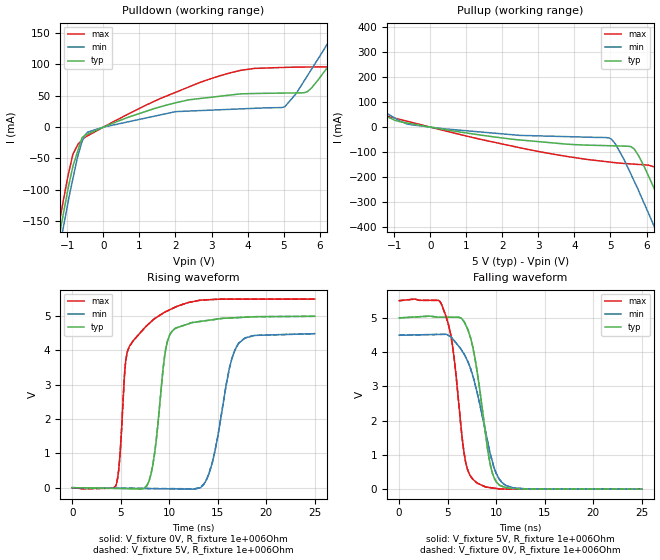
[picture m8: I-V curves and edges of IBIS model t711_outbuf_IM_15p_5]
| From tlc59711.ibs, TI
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|   t711_outbuf 5V Model with
|   1M ohm and 15 pf load during VT transient
[Model] t711_outbuf_IM_15p_5
Model_type   Output
Polarity   Non-Inverting
Vmeas = 2.5
Vref = 2.5
Cref = 15pF
Rref = 50
|   typ   min   max
|   (nom PVT)   (Fast PVT)   (slow PVT)
|   ON state : BUFFER OUTPUT TURNED HIGH
C_comp   1.98646E-12   1.61466E-12   2.27029E-12
|   OFF state: BUFFER OUTPUT TURNED LOW
|C_comp   1.92343E-12   1.92343E-12   1.92343E-12
| Where   nom PVT is  Nominal Process, 5V, 90C
|   Fast PVT is Strong Process, 4.5V, -40C
|   Slow PVT is Weak Process, 5.5V, 150C
|   C_comp - from L-C Tank method, L = 1nH, peak frequency
| variable   typ   min   max
[Voltage Range]   5   4.5   5.5
|Operating Temperature Range
|   25   85   -40
|Junction Temperature Range
[Temperature Range]   90   150   -40
[Pullup Reference]   5   4.5   5.5
[Pulldown Reference]   0   0   0
[Power Clamp Reference]   5   4.5   5.5
[GND Clamp Reference]   0   0   0
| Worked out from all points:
|   slope of the pulldown table from 0 to 0.75 V, typ, clamps not added: 44.2 ohm
|   slope of the pullup table from 0 to 0.75 V, typ, clamps not added: 42.1 ohm
|   falling waveform, V_fixture 5V, R_fixture 1e+006Ohm: 20-80 % time 1.52ns typ, 2.26ns min, 1.29ns max; typ from 5 V to 0.001 V
|   rising waveform, V_fixture 0V, R_fixture 1e+006Ohm: 20-80 % time 1.13ns typ, 1.72ns min, 1.69ns max; typ from 0.001 V to 5 V
|   rising waveform, V_fixture 5V, R_fixture 1e+006Ohm: 20-80 % time 1.13ns typ, 1.73ns min, 1.69ns max; typ from 0.001 V to 5 V
|   falling waveform, V_fixture 0V, R_fixture 1e+006Ohm: 20-80 % time 1.52ns typ, 2.26ns min, 1.29ns max; typ from 5 V to 0.001 V
[Pulldown]
|   Voltage   I(typ)   I(min)   I(max)
-5V       -1.595A    -1.55A     -1.658A
-1.243V   -178.9mA   -200.3mA   -159.4mA
-1.11V    -138mA     -159.3mA   -116.4mA
-840.5mV  -61.25mA   -80.66mA   -42.53mA
-598.2mV  -17.61mA   -23.71mA   -21.08mA
-419.1mV  -10.56mA   -7.658mA   -13.18mA
2.678V    45.63mA    26.39mA    71.32mA
5.023V    54.34mA    32.3mA     95.27mA
5.663V    56.68mA    82.24mA    95.89mA
6.506V    119.4mA    161mA      104mA
7.553V    207mA      262.9mA    172mA
9.985V    423.5mA    510mA      347.6mA
[Pullup]
|   Voltage   I(typ)   I(min)   I(max)
-5V       352.5mA    416.3mA    271.4mA
-2.121V   116.7mA    142.1mA    82.16mA
-663.7mV  17.22mA    13.61mA    24.41mA
2.374V    -49.89mA   -31.61mA   -79mA
4.987V    -74.39mA   -44.7mA    -139.8mA
5.137V    -74.98mA   -67.29mA   -142.3mA
5.663V    -88.31mA   -217.5mA   -148.1mA
6.226V    -250mA     -402.2mA   -159.9mA
6.358V    -295.2mA   -447.7mA   -174.7mA
6.712V    -419.1mA   -571.8mA   -288.4mA
7.056V    -542.9mA   -693.1mA   -417.9mA
9.985V    -1.675A    -1.779A    -1.611A
[Ramp]
R_load = 1e+006
|   typ   min   max
dV/dt_r   2.99723/1.12305e-009   2.69349/1.71464e-009   3.29883/1.66828e-009
dV/dt_f   2.99729/1.51327e-009   2.694/2.23482e-009   3.29884/1.28364e-009
[Falling Waveform]
V_fixture = 5V
V_fixture_min = 4.5V
V_fixture_max = 5.5V
R_fixture = 1e+006Ohm
C_fixture = 0F
|   Time   V(typ)   V(min)   V(max)
0s        4.997V     4.492V     5.499V
4.395ns   5.017V     4.517V     5.376V
5.478ns   5.017V     4.401V     4.233V
6.828ns   4.811V     3.872V     829.5mV
7.406ns   4.372V     3.48V      364.7mV
7.958ns   3.576V     2.908V     195.9mV
9.425ns   680mV      1.002V     44.14mV
10.35ns   116.7mV    284.3mV    7.841mV
13.01ns   7.406mV    10.26mV    4.965mV
25ns      1.236mV    1.639mV    781uV
[Rising Waveform]
V_fixture = 0V
V_fixture_min = 0V
V_fixture_max = 0V
R_fixture = 1e+006Ohm
C_fixture = 0F
|   Time   V(typ)   V(min)   V(max)
0s        980.5uV    1.27mV     592.3uV
4.473ns   -20.11mV   -13.87mV   45.37mV
4.863ns   -21.95mV   -15.19mV   757.9mV
5.641ns   -25.62mV   -17.82mV   3.922V
8.381ns   803.3mV    -27.09mV   4.904V
9.64ns    4.046V     -31.35mV   5.131V
10.6ns    4.641V     -34.59mV   5.26V
13.88ns   4.873V     253.2mV    5.477V
17.2ns    4.96V      4.221V     5.496V
25ns      4.996V     4.49V      5.499V
[Rising Waveform]
V_fixture = 5V
V_fixture_min = 4.5V
V_fixture_max = 5.5V
R_fixture = 1e+006Ohm
C_fixture = 0F
|   Time   V(typ)   V(min)   V(max)
0s        1.236mV    1.637mV    781uV
4.473ns   -17.7mV    -10.1mV    46.4mV
4.863ns   -19.36mV   -11.13mV   759.8mV
5.641ns   -22.65mV   -13.17mV   3.923V
8.381ns   810.4mV    -20.36mV   4.905V
9.64ns    4.05V      -23.66mV   5.132V
10.6ns    4.643V     -26.17mV   5.26V
13.88ns   4.874V     266mV      5.477V
17.2ns    4.961V     4.225V     5.497V
25ns      4.997V     4.491V     5.499V
[Falling Waveform]
|Gnd
V_fixture = 0V
V_fixture_min = 0V
V_fixture_max = 0V
R_fixture = 1e+006Ohm
C_fixture = 0F
|   Time   V(typ)   V(min)   V(max)
0s        4.996V     4.491V     5.499V
4.395ns   5.017V     4.516V     5.375V
5.478ns   5.016V     4.4V       4.232V
6.828ns   4.81V      3.87V      828.1mV
7.406ns   4.37V      3.477V     364mV
7.958ns   3.573V     2.904V     195.4mV
9.425ns   676.9mV    997.3mV    43.79mV
10.35ns   115.7mV    282mV      7.532mV
12.99ns   6.933mV    9.795mV    4.688mV
25ns      980.5uV    1.273mV    592.3uV
